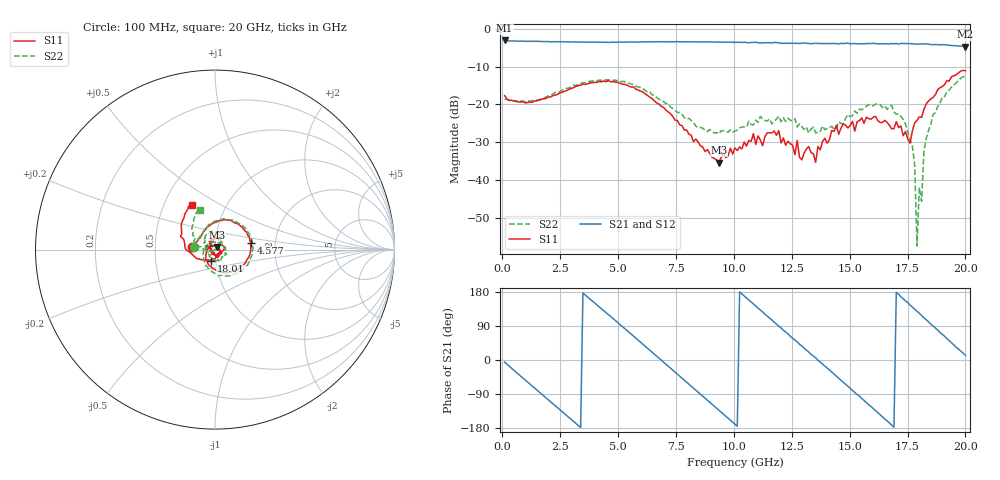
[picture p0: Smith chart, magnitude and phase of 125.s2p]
!Agilent Technologies,N5230C,MY49001569,A.09.33.09
!Agilent N5230C: A.09.33.09
!Date: Tuesday, July 28, 2015 11:12:23
!Correction: S11(Full 2 Port(1,2))
!S21(Full 2 Port(1,2))
!S12(Full 2 Port(1,2))
!S22(Full 2 Port(1,2))
!S2P File: Measurements: S11, S21, S12, S22:
# Hz S  dB  R 50
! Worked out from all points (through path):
!   201 points, 100 MHz to 20 GHz, reference 50 ohm
!   highest |S21| = -3.08 dB at 100 MHz (marker M1); lowest = -4.7 dB at 20 GHz (marker M2)
!   group delay of S21, straight-line fit = 148 ps
!   lowest |S11| = -35.4 dB at 9.354 GHz (marker M3), VSWR 1.03, Z = 51 + j1.42 ohm
!   |S11| at or under -10 dB: start of sweep to end of sweep
!   |S22| runs from -57.4 to -12.5 dB; largest |S21 - S12| = 0.022
!   S11 on the Smith chart (normalised r, x): 100 MHz: 0.77, +0.03; 4.577 GHz: 1.50, +0.12; 18.01 GHz: 0.95, -0.12; 20 GHz: 0.69, +0.37
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1e8  -17.67 172.5  -3.08 -5.7  -3.11 -6.1  -18.67 173.1
1.692e9  -18.65 124.0  -3.37 -89.9  -3.36 -90.0  -18.42 122.4
3.483e9  -14.62 59.4  -3.50 176.7  -3.51 176.8  -14.26 57.5
4.5775e9  -13.69 10.8  -3.61 119.9  -3.58 119.8  -13.52 8.1
5.5725e9  -15.39 -37.6  -3.48 68.1  -3.49 67.9  -14.62 -41.8
6.7665e9  -19.88 -99.5  -3.44 5.0  -3.46 4.8  -18.61 -101.7
8.06e9  -27.82 179.0  -3.42 -64.2  -3.47 -64.2  -23.68 -177.4
9.3535e9  -35.39 55.0  -3.48 -133.0  -3.53 -132.8  -27.79 86.9
1.005e10  -31.49 5.4  -3.58 -169.8  -3.61 -170.0  -27.03 37.6
1.1841e10  -28.14 -65.1  -3.63 94.8  -3.74 94.8  -23.85 -55.9
1.3433e10  -32.99 -158.4  -3.87 10.3  -3.96 9.5  -25.95 -151.0
1.4428e10  -25.47 119.6  -3.90 -42.6  -3.90 -42.1  -26.27 163.7
1.5224e10  -27.06 104.8  -3.90 -85.5  -3.98 -85.1  -21.73 136.4
1.67165e10  -25.49 45.4  -4.00 -166.0  -3.99 -165.9  -20.63 77.0
1.77115e10  -26.92 -82.3  -3.98 139.4  -4.02 139.1  -31.12 23.5
1.7811e10  -24.87 -95.5  -4.02 134.2  -4.13 133.6  -36.15 12.0
1.79105e10  -24.21 -112.1  -4.05 128.4  -4.07 128.6  -57.44 -73.0
1.801e10  -23.26 -107.8  -4.03 123.1  -3.99 122.3  -41.95 43.8
1.81095e10  -23.41 -124.5  -3.99 117.6  -4.18 117.4  -45.58 -135.0
1.8209e10  -21.24 -136.6  -4.04 111.0  -4.11 111.8  -32.34 -156.0
1.8607e10  -18.13 -164.3  -4.17 89.9  -4.15 89.5  -22.61 175.3
2e10  -11.09 117.1  -4.72 12.6  -4.72 11.3  -12.48 110.1
